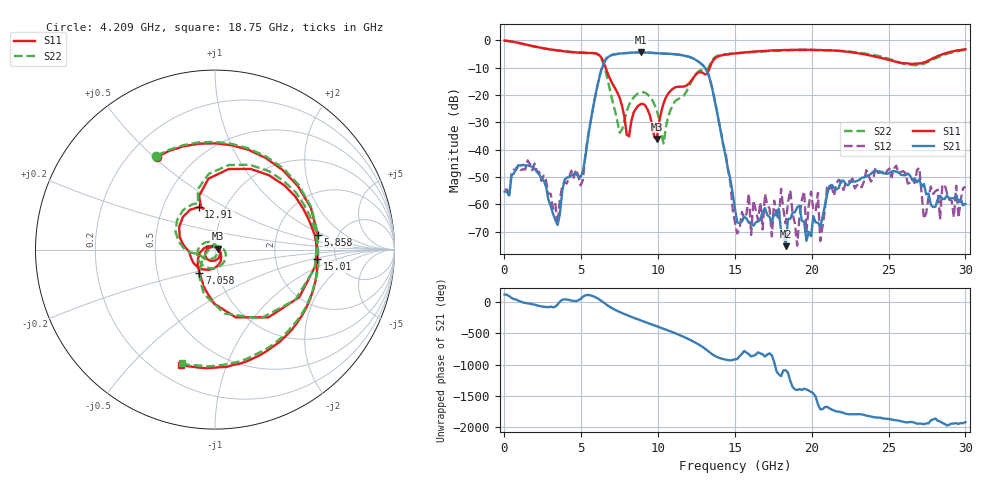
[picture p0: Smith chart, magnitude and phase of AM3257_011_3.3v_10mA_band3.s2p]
!Keysight Technologies,N5245B,MY58422270,A.16.20.02
!Date: Wednesday, June 18, 2025 22:21:49
!Correction: S11(C  2-Port  )
!S21(C  2-Port  )
!S12(C  2-Port  )
!S22(C  2-Port  )
!S2P File: Measurements: S11, S21, S12, S22:
# Hz S  dB  R 50
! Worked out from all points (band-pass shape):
!   201 points, 10 MHz to 30 GHz, reference 50 ohm
!   highest |S21| = -4.44 dB at 8.857 GHz (marker M1); lowest = -75.3 dB at 18.3 GHz (marker M2)
!   |S21| within 3 dB of the highest: 6.565 GHz to 12.52 GHz (5.952 GHz wide, 62.4 % of centre)
!   lowest |S11| = -36.1 dB at 9.907 GHz (marker M3), VSWR 1.03, Z = 51.5 + j0.623 ohm
!   |S11| at or under -10 dB: 6.581 GHz to 13.36 GHz (6.784 GHz wide, 68 % of centre)
!   |S22| runs from -37.8 to -0.1 dB; largest |S21 - S12| = 0.013
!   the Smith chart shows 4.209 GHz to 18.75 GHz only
!   S11 on the Smith chart (normalised r, x): 4.209 GHz: 0.31, +0.51; 5.858 GHz: 3.50, +0.87; 7.058 GHz: 0.81, -0.21; 12.91 GHz: 0.75, +0.38; 15.01 GHz: 3.59, -0.55; 18.75 GHz: 0.30, -0.70
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1e7  -0.18 -1.4  -55.31 114.4  -54.58 -171.0  -0.09 -0.9
1.2096e9  -1.36 -87.7  -45.54 -11.8  -47.18 -14.5  -1.36 -87.6
3.45885e9  -3.75 157.8  -67.52 -44.8  -67.42 -7.3  -3.72 157.4
4.2086e9  -4.29 122.1  -50.14 29.1  -50.02 9.9  -4.20 122.0
5.1083e9  -4.63 71.4  -47.88 79.4  -51.04 81.9  -4.53 71.6
5.85805e9  -4.76 8.3  -21.97 79.1  -21.88 79.6  -4.73 8.0
7.05765e9  -16.20 -124.2  -5.31 -110.9  -5.28 -111.6  -22.76 -147.2
8.1073e9  -35.16 13.7  -4.63 133.8  -4.63 133.8  -23.64 -21.9
8.85705e9  -23.37 -114.0  -4.44 63.7  -4.43 63.7  -19.09 -115.6
9.9067e9  -36.10 22.7  -4.74 -30.0  -4.75 -29.9  -25.44 126.4
1.005665e10  -30.17 -20.1  -4.80 -43.2  -4.79 -43.1  -28.77 105.6
1.14062e10  -17.02 -158.0  -5.33 -171.5  -5.33 -171.4  -21.29 -157.7
1.29057e10  -11.91 110.9  -9.12 -1.5  -9.05 -0.7  -10.99 116.6
1.5005e10  -4.83 -5.2  -61.70 163.0  -66.66 168.5  -4.80 -1.6
1.83039e10  -3.56 -97.7  -75.29 -9.5  -67.02 132.4  -3.73 -96.6
1.875375e10  -3.50 -106.6  -63.08 81.5  -63.45 59.0  -3.61 -105.9
2.01033e10  -3.53 -133.4  -64.31 -19.2  -62.11 -48.5  -3.59 -133.2
2.055315e10  -3.59 -142.2  -68.26 86.7  -73.42 126.0  -3.63 -142.1
2.505165e10  -7.22 93.8  -48.47 -68.9  -46.91 -65.5  -6.84 101.0
2.7001e10  -8.48 -2.0  -50.88 -140.7  -46.62 -130.7  -8.89 2.6
2.73009e10  -8.15 -13.3  -52.56 -151.1  -65.28 -139.3  -8.67 -9.1
3e10  -3.33 -97.1  -59.81 -116.6  -53.58 -97.6  -3.52 -99.2
